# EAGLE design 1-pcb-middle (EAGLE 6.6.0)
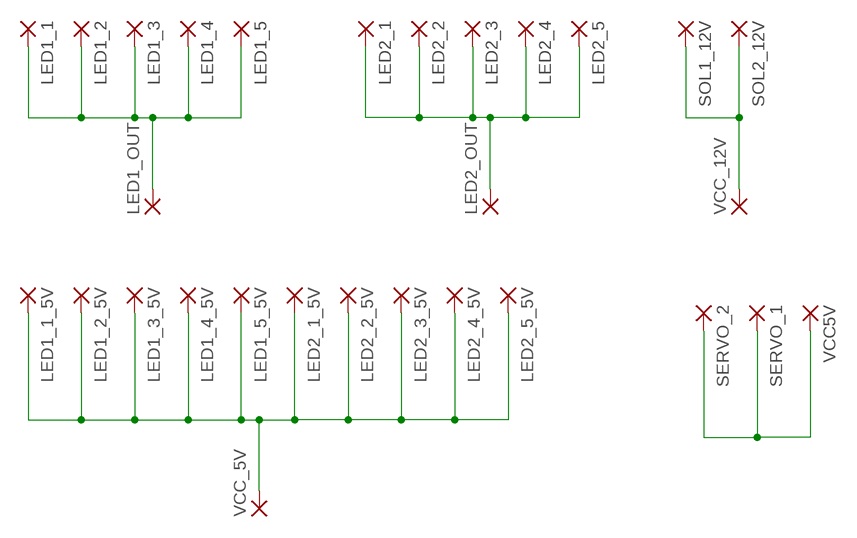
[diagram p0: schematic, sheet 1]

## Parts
LED1_1  2,15/1,0  [2,15/1,0]
LED1_1_5V  2,15/1,0  [2,15/1,0]
LED1_2  2,15/1,0  [2,15/1,0]
LED1_2_5V  2,15/1,0  [2,15/1,0]
LED1_3  2,15/1,0  [2,15/1,0]
LED1_3_5V  2,15/1,0  [2,15/1,0]
LED1_4  2,15/1,0  [2,15/1,0]
LED1_4_5V  2,15/1,0  [2,15/1,0]
LED1_5  2,15/1,0  [2,15/1,0]
LED1_5_5V  2,15/1,0  [2,15/1,0]
LED1_OUT  2,15/1,0  [2,15/1,0]
LED2_1  2,15/1,0  [2,15/1,0]
LED2_1_5V  2,15/1,0  [2,15/1,0]
LED2_2  2,15/1,0  [2,15/1,0]
LED2_2_5V  2,15/1,0  [2,15/1,0]
LED2_3  2,15/1,0  [2,15/1,0]
LED2_3_5V  2,15/1,0  [2,15/1,0]
LED2_4  2,15/1,0  [2,15/1,0]
LED2_4_5V  2,15/1,0  [2,15/1,0]
LED2_5  2,15/1,0  [2,15/1,0]
LED2_5_5V  2,15/1,0  [2,15/1,0]
LED2_OUT  2,15/1,0  [2,15/1,0]
SERVO_1  2,15/1,0  [2,15/1,0]
SERVO_2  2,15/1,0  [2,15/1,0]
SOL1_12V  2,15/1,0  [2,15/1,0]
SOL2_12V  2,15/1,0  [2,15/1,0]
VCC5V  2,15/1,0  [2,15/1,0]
VCC_5V  2,15/1,0  [2,15/1,0]
VCC_12V  2,15/1,0  [2,15/1,0]

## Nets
N$1: LED1_1.1(P) LED1_2.1(P) LED1_3.1(P) LED1_4.1(P) LED1_5.1(P) LED1_OUT.1(P)
N$2: LED1_1_5V.1(P) LED1_2_5V.1(P) LED1_3_5V.1(P) LED1_4_5V.1(P) LED1_5_5V.1(P) LED2_1_5V.1(P) LED2_2_5V.1(P) LED2_3_5V.1(P) LED2_4_5V.1(P) LED2_5_5V.1(P) VCC_5V.1(P)
N$3: SOL1_12V.1(P) SOL2_12V.1(P) VCC_12V.1(P)
N$4: SERVO_1.1(P) SERVO_2.1(P) VCC5V.1(P)
N$5: LED2_1.1(P) LED2_2.1(P) LED2_3.1(P) LED2_4.1(P) LED2_5.1(P) LED2_OUT.1(P)

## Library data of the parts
LED1_1 LED1_1_5V LED1_2 LED1_2_5V LED1_3 LED1_3_5V LED1_4 LED1_4_5V LED1_5 LED1_5_5V LED1_OUT LED2_1 LED2_1_5V LED2_2 LED2_2_5V LED2_3 LED2_3_5V LED2_4 LED2_4_5V LED2_5 LED2_5_5V LED2_OUT SERVO_1 SERVO_2 SOL1_12V SOL2_12V VCC5V VCC_5V VCC_12V = wirepad:2,15/1,0: THROUGH-HOLE PAD

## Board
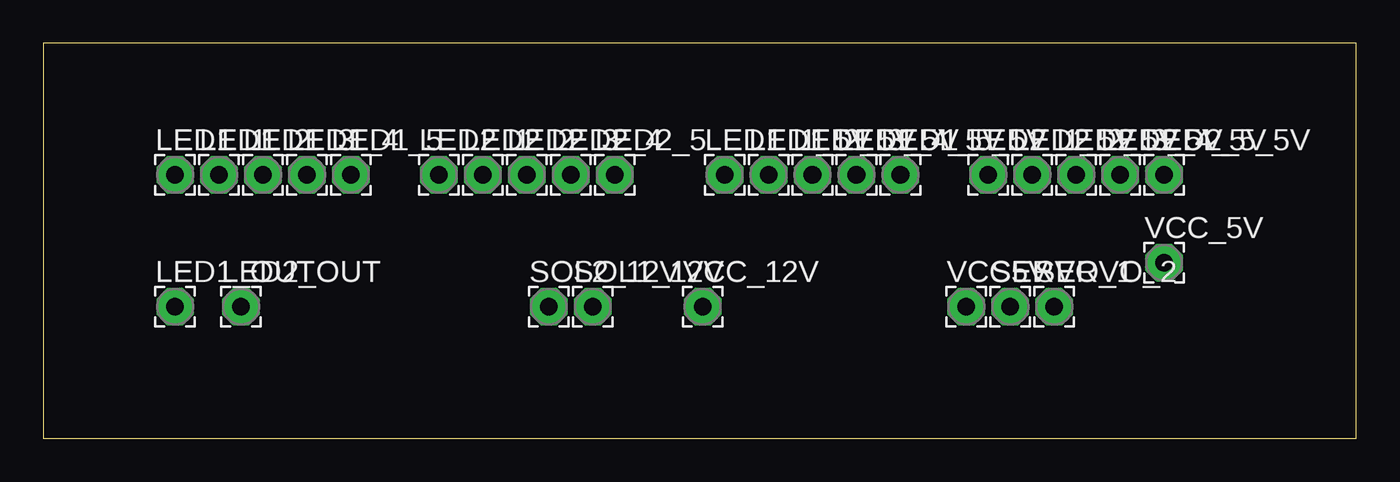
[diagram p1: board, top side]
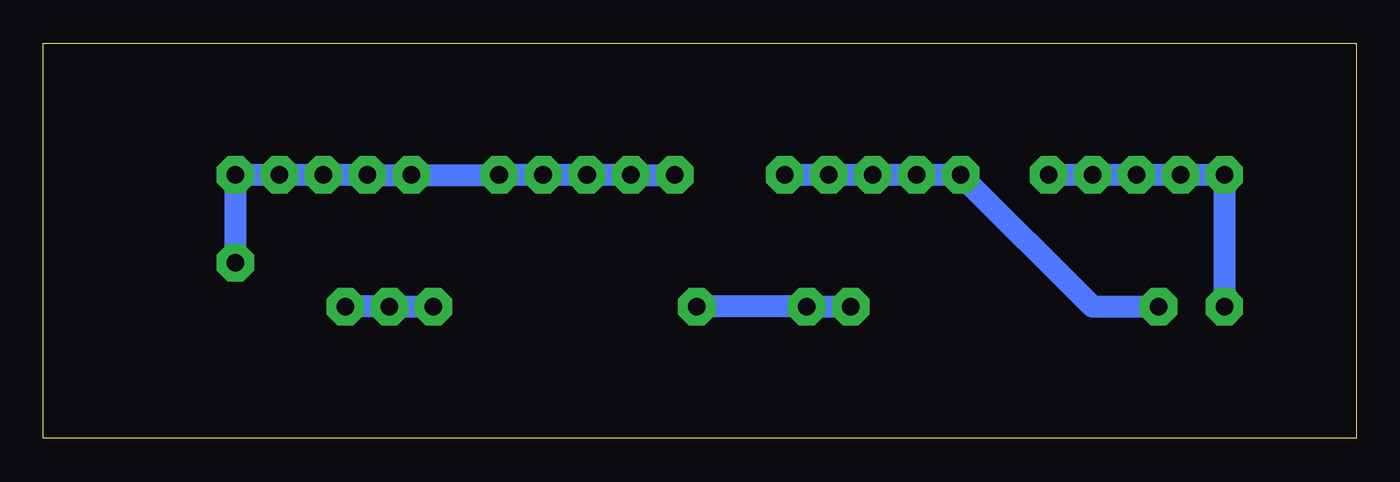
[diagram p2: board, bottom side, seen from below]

Size 75.87 x 22.85 mm. Coordinates in mm from the lower left corner, seen from the top.
Outline: 0,0 75.87,0 75.87,22.85 0,22.85 0,0
Copper layers (1*16): Top 0.035mm / dielectric 1.5mm / Bottom 0.035mm
Design rules "default": minimum track width 10mil, minimum drill 24mil, track to track 8mil, track to pad 8mil, pad to pad 8mil, via to via 8mil, smd to smd 8mil, copper to edge 40mil, drill to drill 8mil, minimum pad ring 10mil, minimum via ring 8mil, stop-mask expansion 4mil, vias tented up to drill 0mil, thermal gap 10mil

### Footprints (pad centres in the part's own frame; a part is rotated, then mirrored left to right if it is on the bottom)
2,15/1,0 = drill 1.016 pad 2.159 octagon: 1 0,0

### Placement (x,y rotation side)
LED1_1  7.62,15.24 0 top
LED1_1_5V  39.37,15.24 0 top
LED1_2  10.16,15.24 0 top
LED1_2_5V  41.91,15.24 0 top
LED1_3  12.7,15.24 0 top
LED1_3_5V  44.45,15.24 0 top
LED1_4  15.24,15.24 0 top
LED1_4_5V  46.99,15.24 0 top
LED1_5  17.78,15.24 0 top
LED1_5_5V  49.53,15.24 0 top
LED1_OUT  7.62,7.62 0 top
LED2_1  22.86,15.24 0 top
LED2_1_5V  54.61,15.24 0 top
LED2_2  25.4,15.24 0 top
LED2_2_5V  57.15,15.24 0 top
LED2_3  27.94,15.24 0 top
LED2_3_5V  59.69,15.24 0 top
LED2_4  30.48,15.24 0 top
LED2_4_5V  62.23,15.24 0 top
LED2_5  33.02,15.24 0 top
LED2_5_5V  64.77,15.24 0 top
LED2_OUT  11.43,7.62 0 top
SERVO_1  55.88,7.62 0 top
SERVO_2  58.42,7.62 0 top
SOL1_12V  31.75,7.62 0 top
SOL2_12V  29.21,7.62 0 top
VCC5V  53.34,7.62 0 top
VCC_5V  64.77,10.16 0 top
VCC_12V  38.1,7.62 0 top

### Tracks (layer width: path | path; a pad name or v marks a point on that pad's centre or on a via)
N$1
  Bottom 1.27: LED1_OUT.1 LED1_1.1 LED1_2.1 LED1_3.1 LED1_4.1 LED1_5.1
N$2
  Bottom 1.27: LED1_1_5V.1 LED1_2_5V.1 LED1_3_5V.1 LED1_4_5V.1 LED1_5_5V.1 LED2_1_5V.1 LED2_2_5V.1 LED2_3_5V.1 LED2_4_5V.1 LED2_5_5V.1 VCC_5V.1
N$3
  Bottom 1.27: SOL2_12V.1 SOL1_12V.1 VCC_12V.1
N$4
  Bottom 1.27: VCC5V.1 SERVO_1.1 SERVO_2.1
N$5
  Bottom 1.27: LED2_OUT.1 15.24,7.62 LED2_1.1 LED2_2.1 LED2_3.1 LED2_4.1 LED2_5.1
